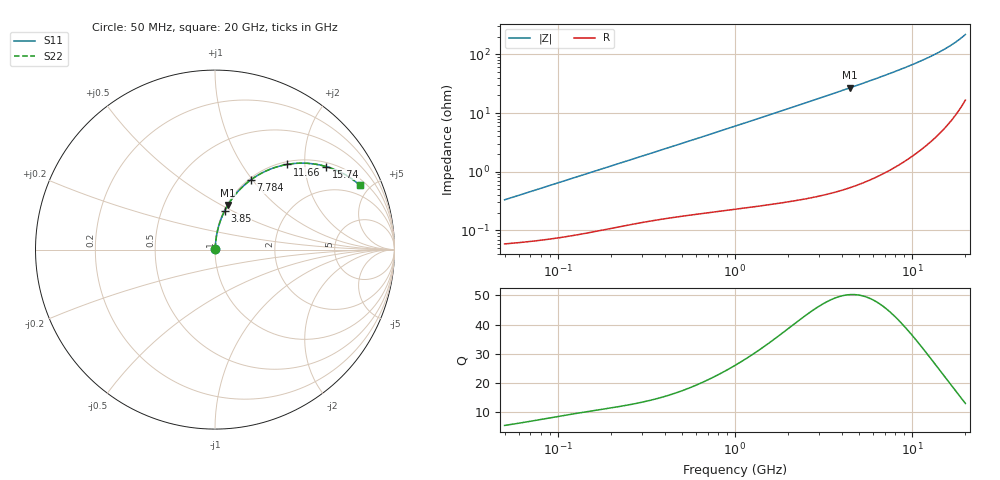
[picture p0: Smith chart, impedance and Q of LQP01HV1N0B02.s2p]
!Murata Part Number: LQP01HV1N0B02
!These Parameters are Measured in Series Mode Connection
!  o--[Z]--o
!Port1  Port2
!  o-------o
!Freq. Start=50[MHz] Stop=20[GHz], 401[Steps]
# Hz S RI R 50
!Freq.(Hz) S11(Real) S11(Imag) S21(Real) S21(Imag) S12(Real) S12(Imag) S22(Real) S22(Imag)
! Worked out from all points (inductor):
!   401 points, 50 MHz to 20 GHz, reference 50 ohm
!   read as one part in series: L = 1.04 nH near 51.52 MHz
!   highest Q = 50.2 at 4.472 GHz (marker M1), where L = 959 pH
!   S11 on the Smith chart (normalised r, x): 50 MHz: 1.00, +0.01; 3.85 GHz: 1.01, +0.46; 7.784 GHz: 1.02, +0.98; 11.66 GHz: 1.05, +1.62; 15.74 GHz: 1.12, +2.58; 20 GHz: 1.33, +4.34
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5e7  0.000601 0.00327  0.9994 -0.00327  0.9994 -0.00327  0.000601 0.00327
5.30873e7  0.000611 0.00347  0.9994 -0.00347  0.9994 -0.00347  0.000611 0.00347
1.364002e8  0.000945 0.00866  0.9991 -0.00866  0.9991 -0.00866  0.000945 0.00866
3.721004e8  0.00204 0.0227  0.998 -0.0227  0.998 -0.0227  0.00204 0.0227
6.380365e8  0.00338 0.0382  0.9966 -0.0382  0.9966 -0.0382  0.00338 0.0382
1e9  0.00581 0.0592  0.9942 -0.0592  0.9942 -0.0592  0.00581 0.0592
1.714689e9  0.013 0.1002  0.987 -0.1002  0.987 -0.1002  0.013 0.1002
2.728004e9  0.029 0.157  0.971 -0.157  0.971 -0.157  0.029 0.157
3.850025e9  0.0544 0.217  0.9456 -0.217  0.9456 -0.217  0.0544 0.217
4.472136e9  0.072 0.2486  0.928 -0.2486  0.928 -0.2486  0.072 0.2486
5.856089e9  0.1189 0.3136  0.8811 -0.3136  0.8811 -0.3136  0.1189 0.3136
7.442007e9  0.1847 0.377  0.8153 -0.377  0.8153 -0.377  0.1847 0.377
7.784049e9  0.2004 0.3889  0.7996 -0.3889  0.7996 -0.3889  0.2004 0.3889
8.644534e9  0.2416 0.4159  0.7584 -0.4159  0.7584 -0.4159  0.2416 0.4159
9.600142e9  0.29 0.4407  0.71 -0.4407  0.71 -0.4407  0.29 0.4407
1.066139e10  0.3463 0.4614  0.6537 -0.4614  0.6537 -0.4614  0.3463 0.4614
1.166392e10  0.4009 0.4744  0.5991 -0.4744  0.5991 -0.4744  0.4009 0.4744
1.375312e10  0.5157 0.4808  0.4843 -0.4808  0.4843 -0.4808  0.5157 0.4808
1.573793e10  0.6203 0.4623  0.3797 -0.4623  0.3797 -0.4623  0.6203 0.4623
1.747767e10  0.7043 0.4289  0.2957 -0.4289  0.2957 -0.4289  0.7043 0.4289
1.940974e10  0.7856 0.3764  0.2144 -0.3764  0.2144 -0.3764  0.7856 0.3764
2e10  0.8076 0.3578  0.1924 -0.3578  0.1924 -0.3578  0.8076 0.3578
